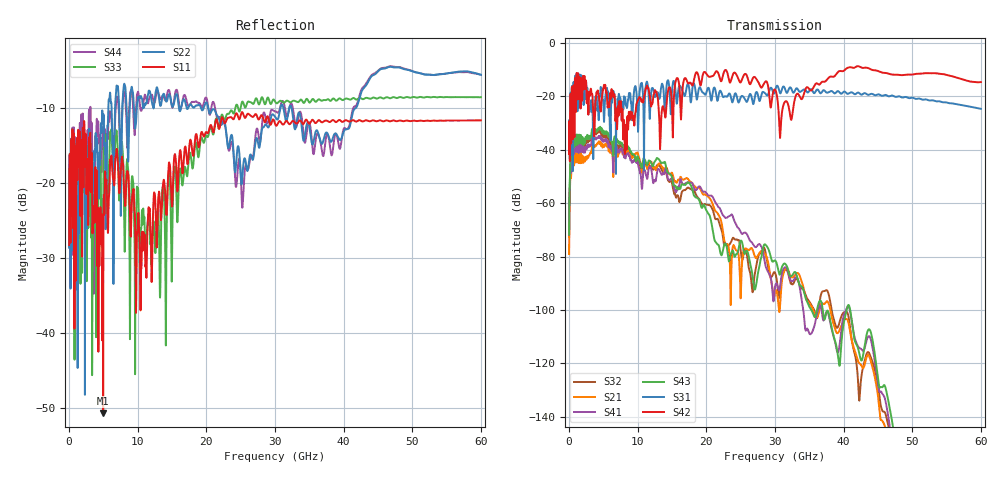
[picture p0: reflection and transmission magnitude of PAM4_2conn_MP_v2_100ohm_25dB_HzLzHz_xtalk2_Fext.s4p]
! Info: Touchstone file created by Circ.  Input file=FAB50GbE_2conn_Midplane_Examax_Topo2_v2_100ohm_25dB_HzLzHz.circ
# Hz S RI R 50
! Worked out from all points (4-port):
!   6000 points, 10 MHz to 60 GHz, reference 50 ohm
!   strongest paths, dB at 10 MHz, 15.01 GHz, 30.01 GHz, 45.01 GHz, 60 GHz:
!     S42: -41.6, -24.7, -17.5, -10.5, -14.7
!     S31: -41.2, -17.6, -17.9, -19.3, -24.7
!     S43: -71.8, -50.4, -81.5, -125.6, -173.7
!     S41: -71.8, -50.3, -91.4, -127.7, -184.2
!     S21: -79.1, -48.7, -93.4, -132.2, -179.3
!     S32: -72.6, -52.5, -86.1, -128.0, -176.6
!   lowest |S11| = -50.6 dB at 4.97 GHz (marker M1), VSWR 1.01, Z = 50.2 - j0.171 ohm
!   |S11| at or under -10 dB: start of sweep to end of sweep
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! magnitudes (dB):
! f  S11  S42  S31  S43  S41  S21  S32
! 10 MHz  -28.2  -41.6  -41.2  -71.8  -71.8  -79.1  -72.6
! 830 MHz  -19.3  -17.3  -14.9  -34.8  -36.8  -40.2  -36.5
! 4.97 GHz  -50.6  -17.5  -21.6  -32.7  -36.1  -38.1  -34.1
! 8.15 GHz  -22.7  -39.2  -20.4  -39.7  -42.7  -41.9  -40.6
! 23.36 GHz  -11.2  -14.6  -18.9  -81.5  -64.9  -79.2  -75.5
! 30.8 GHz  -11.8  -33.6  -18.9  -86.1  -90.3  -95.6  -91.2
! 60 GHz  -11.6  -14.7  -24.7  -173.7  -184.2  -179.3  -176.6
